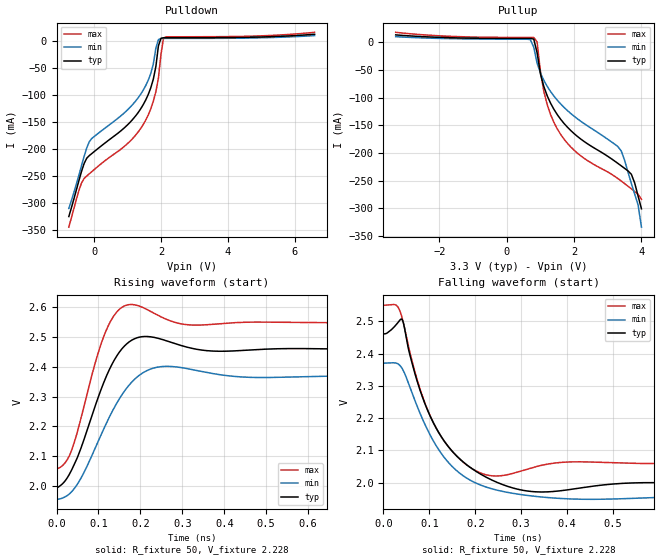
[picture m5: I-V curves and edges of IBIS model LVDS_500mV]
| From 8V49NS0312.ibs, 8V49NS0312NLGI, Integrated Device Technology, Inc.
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[Model]   LVDS_500mV
Model_type   Output
Polarity   Non-Inverting
|   typ   min   max
C_comp   2pF   1.5pF   2.5pF
Vmeas = 2.252V
Rref = 50
Cref = 0
Vref = 2.252V
|   typ   min   max
[Voltage range]   3.3V   3.135V   3.465V
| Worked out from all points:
|   slope of the pulldown table from 0 to 0.495 V, typ, clamps not added: 20.7 ohm
|   slope of the pullup table from 0 to 0.495 V, typ, clamps not added: 10.3 kohm
|   rising waveform, R_fixture 50, V_fixture 2.228: 20-80 % time 70.8ps typ, 84.2ps min, 55.6ps max; typ from 2 V to 2.46 V
|   falling waveform, R_fixture 50, V_fixture 2.228: 20-80 % time 91.9ps typ, 98.1ps min, 69.2ps max; typ from 2.46 V to 2 V
[Pulldown]
|Voltage   I (typ)   I (min)   I (max)
|Note, modeling breaks down at 250mA and above.  This is well beyond the functional   |
|operating range of the device.  Should this scenario occur, catastrophic failure and   |
|possible damage to the device and/or board is of higher concern than the I-V curve   |
|behavior.  The IBIS checker will flag currents in excess of 10A with warnings.  Lines   |
|with currents in excess of 0.35 A have been commented out.  The points still remain|
|available to the user if the user desires to use them.   |
|-1.00000e+00   -4.13253e-01   -4.09298e-01   -4.19390e-01
|-9.23232e-01   -3.67552e-01   -3.68435e-01   -3.77970e-01
|-8.46465e-01   -3.40305e-01   -3.28212e-01   -3.60598e-01
-769.7mV  -324.3mA   -309.3mA   -343.8mA
-385.9mV  -240.1mA   -229.3mA   -261.8mA
-155.6mV  -211.3mA   -185.5mA   -245mA
996mV     -154.1mA   -126.3mA   -188.8mA
1.533V    -108.7mA   -82.08mA   -145.9mA
1.687V    -85.96mA   -59.43mA   -125mA
1.764V    -69.91mA   -41.89mA   -111mA
1.84V     -46.51mA   -12.56mA   -93.07mA
1.917V    -8.142mA   3.4mA      -67.78mA
1.994V    5.882mA    5.534mA    -23.91mA
2.071V    6.864mA    5.691mA    6.534mA
6.6V      13.37mA    10.91mA    16.96mA
[Pullup]
|Voltage   I (typ)   I (min)   I (max)
|Note, modeling breaks down at 250mA and above.  This is well beyond the functional   |
|operating range of the device.  Should this scenario occur, catastrophic failure and   |
|possible damage to the device and/or board is of higher concern than the I-V curve   |
|behavior.  The IBIS checker will flag currents in excess of 10A with warnings.  Lines   |
|with currents in excess of 0.35 A have been commented out.  The points still remain|
|available to the user if the user desires to use them.   |
|Note, modeling breaks down at 250mA and above.  This is well beyond the functional   |
|operating range of the device.  Should this scenario occur, catastrophic failure and   |
|possible damage to the device and/or board is of higher concern than the I-V curve   |
|behavior.  The IBIS checker will flag currents in excess of 10A with warnings.  Lines   |
|with currents in excess of 0.35 A have been commented out.  The points still remain|
|available to the user if the user desires to use them.   |
|Note, modeling breaks down at 250mA and above.  This is well beyond the functional   |
|operating range of the device.  Should this scenario occur, catastrophic failure and   |
|possible damage to the device and/or board is of higher concern than the I-V curve   |
|behavior.  The IBIS checker will flag currents in excess of 10A with warnings.  Lines   |
|with currents in excess of 0.35 A have been commented out.  The points still remain|
|available to the user if the user desires to use them.   |
|Note, modeling breaks down at 250mA and above.  This is well beyond the functional   |
|operating range of the device.  Should this scenario occur, catastrophic failure and   |
|possible damage to the device and/or board is of higher concern than the I-V curve   |
|behavior.  The IBIS checker will flag currents in excess of 10A with warnings.  Lines   |
|with currents in excess of 0.35 A have been commented out.  The points still remain|
|available to the user if the user desires to use them.   |
|Note, modeling breaks down at 250mA and above.  This is well beyond the functional   |
|operating range of the device.  Should this scenario occur, catastrophic failure and   |
|possible damage to the device and/or board is of higher concern than the I-V curve   |
|behavior.  The IBIS checker will flag currents in excess of 10A with warnings.  Lines   |
|with currents in excess of 0.35 A have been commented out.  The points still remain|
|available to the user if the user desires to use them.   |
|Note, modeling breaks down at 250mA and above.  This is well beyond the functional   |
|operating range of the device.  Should this scenario occur, catastrophic failure and   |
|possible damage to the device and/or board is of higher concern than the I-V curve   |
|behavior.  The IBIS checker will flag currents in excess of 10A with warnings.  Lines   |
|with currents in excess of 0.35 A have been commented out.  The points still remain|
|available to the user if the user desires to use them.   |
-3.3V     13.37mA    10.15mA    18.01mA
700mV     6.924mA    4.738mA    8.747mA
800mV     5.854mA    -8.72mA    8.654mA
900mV     -18.7mA    -37.78mA   545.3uA
1V        -57.22mA   -55.48mA   -53.09mA
1.2V      -96.63mA   -79.62mA   -112.7mA
1.6V      -139.2mA   -111.4mA   -166.5mA
2.2V      -175mA     -142.9mA   -205.4mA
3.4V      -223.4mA   -196.5mA   -250.7mA
3.7V      -238.6mA   -255.4mA   -264.9mA
3.9V      -278mA     -294mA     -274.8mA
4V        -301.1mA   -334.2mA   -283.8mA
|||||| 4.10000e+00   -3.20992e-01   -3.84916e-01   -3.05246e-01
|||||| 4.20000e+00   -3.44358e-01   -4.35056e-01   -3.30580e-01
|||||| 4.30000e+00   -4.03103e-01   -4.84656e-01   -3.53616e-01
|||||| 4.40000e+00   -4.63450e-01   -5.34051e-01   -3.74781e-01
|||||| 4.50000e+00   -5.23396e-01   -5.83693e-01   -4.35513e-01
|||||| 4.60000e+00   -5.83316e-01   -6.33437e-01   -5.04078e-01
|||||| 4.70000e+00   -6.44205e-01   -6.33437e-01   -5.72355e-01
|||||| 4.80000e+00   -7.05373e-01   -6.33437e-01   -6.40700e-01
|||||| 4.90000e+00   -7.65774e-01   -6.33437e-01   -7.10840e-01
|||||| 5.00000e+00   -8.25549e-01   -6.33437e-01   -7.81965e-01
|||||| 5.10000e+00   -8.84997e-01   -6.33437e-01   -8.52375e-01
|||||| 5.20000e+00   -9.44275e-01   -6.33437e-01   -9.21457e-01
|||||| 5.30000e+00   -9.44275e-01   -6.33437e-01   -9.89673e-01
|||||| 5.40000e+00   -9.44275e-01   -6.33437e-01   -1.05773e+00
|||||| 5.50000e+00   -9.44275e-01   -6.33437e-01   -1.12567e+00
[Ramp]
|   typ   min   max
dV/dt_r   0.304/0.079n   0.268/0.093n   0.33/0.064n
dV/dt_f   0.322/0.105n   0.254/0.102n   0.319/0.082n
R_load =   50.0000
[Rising Waveform]
R_fixture = 50
V_fixture   =2.228  |Vcc_typ
V_fixture_min=2.162  |Vcc_min
V_fixture_max=2.304  |Vcc_max
C_fixture = 0.0p
| Time   typ   min   max
0s        1.995V     1.954V     2.058V
36.04ps   2.053V     1.98V      2.12V
94.09ps   2.276V     2.133V     2.422V
120.1ps   2.373V     2.214V     2.528V
170.2ps   2.481V     2.334V     2.609V
212.2ps   2.502V     2.385V     2.596V
262.3ps   2.488V     2.402V     2.56V
358.4ps   2.455V     2.381V     2.542V
478.5ps   2.458V     2.364V     2.551V
2ns       2.46V      2.369V     2.549V
[Falling Waveform]
R_fixture = 50
V_fixture   =2.228  |Vcc_typ
V_fixture_min=2.162  |Vcc_min
V_fixture_max=2.304  |Vcc_max
C_fixture = 0.0p
| Time   typ   min   max
0s        2.461V     2.37V      2.55V
28.03ps   2.49V      2.371V     2.55V
40.04ps   2.507V     2.356V     2.515V
76.08ps   2.303V     2.228V     2.307V
116.1ps   2.166V     2.112V     2.166V
170.2ps   2.068V     2.025V     2.068V
230.2ps   2.012V     1.983V     2.022V
344.3ps   1.971V     1.955V     2.053V
566.6ps   2V         1.952V     2.059V
2ns       1.997V     1.956V     2.06V
